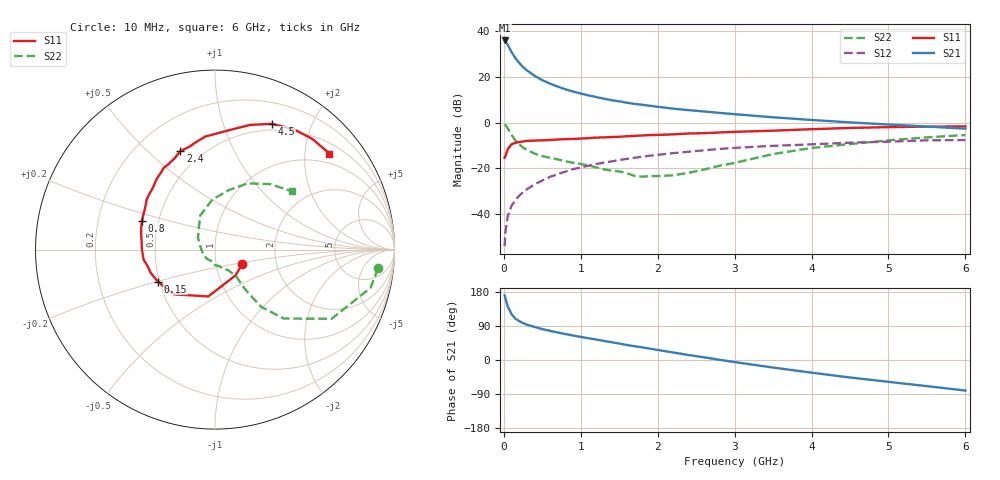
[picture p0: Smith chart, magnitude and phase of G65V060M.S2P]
! SIEMENS Small Signal Semiconductors
! BFG193
! Si NPN RF Bipolar Junction Transistor in SOT223
! VCE = 5 V  IC = 60 mA
! Common Emitter S-Parameters:  August  1996
# GHz  S  MA  R  50
!  f  S11  S21  S12  S22
! GHz  MAG  ANG  MAG  ANG  MAG  ANG  MAG  ANG
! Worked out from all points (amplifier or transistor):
!   36 points, 10 MHz to 6 GHz, reference 50 ohm
!   highest |S21| = 36.0 dB at 10 MHz (marker M1)
!   |S21| within 3 dB of that: start of sweep to 67.33 MHz
!   unconditionally stable (mu >= 1): 404.7 MHz to 2.317 GHz
!   at 250 MHz: K = 0.93, MSG = 27.4 dB, |S12| = -30.4 dB
!   at 1.4 GHz: K = 1.05, MAG = 12.1 dB, |S12| = -16.9 dB
!   at 6 GHz: K = 0.89, MSG = 2.5 dB, |S12| = -7.6 dB
!   S11 on the Smith chart (normalised r, x): 10 MHz: 1.34, -0.22; 150 MHz: 0.49, -0.20; 800 MHz: 0.40, +0.16; 2.4 GHz: 0.38, +0.64; 4.5 GHz: 0.43, +1.47; 6 GHz: 0.74, +2.56
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0.01  0.1725 -27.6  62.94 170.6  0.002 88.5  0.915 -6.6
0.02  0.1837 -52.0  60.31 162.7  0.004 75.4  0.8914 -13.9
0.05  0.2635 -98.1  50.44 141.4  0.009 71.3  0.7553 -30.7
0.1  0.3381 -132.5  35.28 121.4  0.0152 68.9  0.5422 -45.1
0.15  0.3643 -150.6  25.75 109.2  0.0204 68.1  0.4116 -51.0
0.2  0.3802 -159.6  20.28 102.5  0.0254 70.5  0.3394 -52.0
0.25  0.388 -166.8  16.51 97.3  0.0302 70.1  0.2851 -52.7
0.3  0.4016 -172.1  13.95 93.2  0.0351 71.0  0.2558 -52.7
0.4  0.4073 179.9  10.61 87.3  0.045 70.7  0.2114 -52.1
0.5  0.4121 173.0  8.529 81.5  0.0546 69.4  0.1862 -51.5
0.6  0.4202 168.2  7.164 77.0  0.0654 68.5  0.1712 -52.5
0.7  0.4293 163.3  6.168 72.6  0.0752 67.0  0.1578 -54.7
0.8  0.4378 158.4  5.388 68.5  0.0852 65.0  0.1434 -56.4
0.9  0.443 154.8  4.81 64.6  0.0962 63.3  0.1335 -57.8
1.1  0.4601 147.0  3.96 57.5  0.115 59.6  0.1165 -67.0
1.6  0.5065 130.6  2.737 39.6  0.1626 48.8  0.0784 -96.8
2.2  0.5569 113.8  2.034 19.9  0.2163 35.1  0.0708 -161.2
2.4  0.5815 109.4  1.886 13.2  0.2325 30.9  0.0803 172.1
3.5  0.6702 83.2  1.315 -19.9  0.3121 3.8  0.2069 113.6
4.5  0.7693 65.6  1.017 -46.2  0.3666 -16.2  0.3419 76.6
5.5  0.8216 48.5  0.825 -69.0  0.4123 -39.6  0.4778 49.8
6  0.8321 40.0  0.743 -80.6  0.418 -53.0  0.5393 36.9
